{attribute 'qualified_only'}
VAR_GLOBAL

	//FFU
	FFU_ALARM_EN	:	UINT;	//报警输出使能
	FFU_HSPEED		:	UINT;	//转速上限
	FFU_LSPEED		:	UINT;	//转速下限
	
	FFU1_1_POWER_ON	:	UINT	;	//	0:停止，1：运行
	FFU1_2_POWER_ON	:	UINT	;	//	0:停止，1：运行
	FFU1_3_POWER_ON	:	UINT	;	//	0:停止，1：运行
	FFU1_4_POWER_ON	:	UINT	;	//	0:停止，1：运行
	FFU1_5_POWER_ON	:	UINT	;	//	0:停止，1：运行
	FFU1_6_POWER_ON	:	UINT	;	//	0:停止，1：运行
	FFU2_1_POWER_ON	:	UINT	;	//	0:停止，1：运行
	FFU2_2_POWER_ON	:	UINT	;	//	0:停止，1：运行
	FFU2_3_POWER_ON	:	UINT	;	//	0:停止，1：运行
	FFU2_4_POWER_ON	:	UINT	;	//	0:停止，1：运行
	FFU2_5_POWER_ON	:	UINT	;	//	0:停止，1：运行
	FFU2_6_POWER_ON	:	UINT	;	//	0:停止，1：运行
	FFU3_1_POWER_ON	:	UINT	;	//	0:停止，1：运行
	FFU3_2_POWER_ON	:	UINT	;	//	0:停止，1：运行
	FFU3_3_POWER_ON	:	UINT	;	//	0:停止，1：运行
	FFU3_4_POWER_ON	:	UINT	;	//	0:停止，1：运行
	FFU3_5_POWER_ON	:	UINT	;	//	0:停止，1：运行
	FFU3_6_POWER_ON	:	UINT	;	//	0:停止，1：运行

	FFU1_1_SPEED_SV	:	UINT	;	//	FFU1_1设定转速
	FFU1_2_SPEED_SV	:	UINT	;	//	FFU1_2设定转速
	FFU1_3_SPEED_SV	:	UINT	;	//	FFU1_3设定转速
	FFU1_4_SPEED_SV	:	UINT	;	//	FFU1_4设定转速
	FFU1_5_SPEED_SV	:	UINT	;	//	FFU1_5设定转速
	FFU1_6_SPEED_SV	:	UINT	;	//	FFU1_6设定转速
	FFU2_1_SPEED_SV	:	UINT	;	//	FFU2_1设定转速
	FFU2_2_SPEED_SV	:	UINT	;	//	FFU2_2设定转速
	FFU2_3_SPEED_SV	:	UINT	;	//	FFU2_3设定转速
	FFU2_4_SPEED_SV	:	UINT	;	//	FFU2_4设定转速
	FFU2_5_SPEED_SV	:	UINT	;	//	FFU2_5设定转速
	FFU2_6_SPEED_SV	:	UINT	;	//	FFU2_6设定转速
	FFU3_1_SPEED_SV	:	UINT	;	//	FFU3_1设定转速
	FFU3_2_SPEED_SV	:	UINT	;	//	FFU3_2设定转速
	FFU3_3_SPEED_SV	:	UINT	;	//	FFU3_3设定转速
	FFU3_4_SPEED_SV	:	UINT	;	//	FFU3_4设定转速
	FFU3_5_SPEED_SV	:	UINT	;	//	FFU3_5设定转速
	FFU3_6_SPEED_SV	:	UINT	;	//	FFU3_6设定转速

	FFU1_1_EN		:	UINT	;	//	FFU1_1使能
	FFU1_2_EN		:	UINT	;	//	FFU1_2使能
	FFU1_3_EN		:	UINT	;	//	FFU1_3使能
	FFU1_4_EN		:	UINT	;	//	FFU1_4使能
	FFU1_5_EN		:	UINT	;	//	FFU1_5使能
	FFU1_6_EN		:	UINT	;	//	FFU1_6使能
	FFU2_1_EN		:	UINT	;	//	FFU2_1使能
	FFU2_2_EN		:	UINT	;	//	FFU2_2使能
	FFU2_3_EN		:	UINT	;	//	FFU2_3使能
	FFU2_4_EN		:	UINT	;	//	FFU2_4使能
	FFU2_5_EN		:	UINT	;	//	FFU2_5使能
	FFU2_6_EN		:	UINT	;	//	FFU2_6使能
	FFU3_1_EN		:	UINT	;	//	FFU3_1使能
	FFU3_2_EN		:	UINT	;	//	FFU3_2使能
	FFU3_3_EN		:	UINT	;	//	FFU3_3使能
	FFU3_4_EN		:	UINT	;	//	FFU3_4使能
	FFU3_5_EN		:	UINT	;	//	FFU3_5使能
	FFU3_6_EN		:	UINT	;	//	FFU3_6使能

END_VAR
